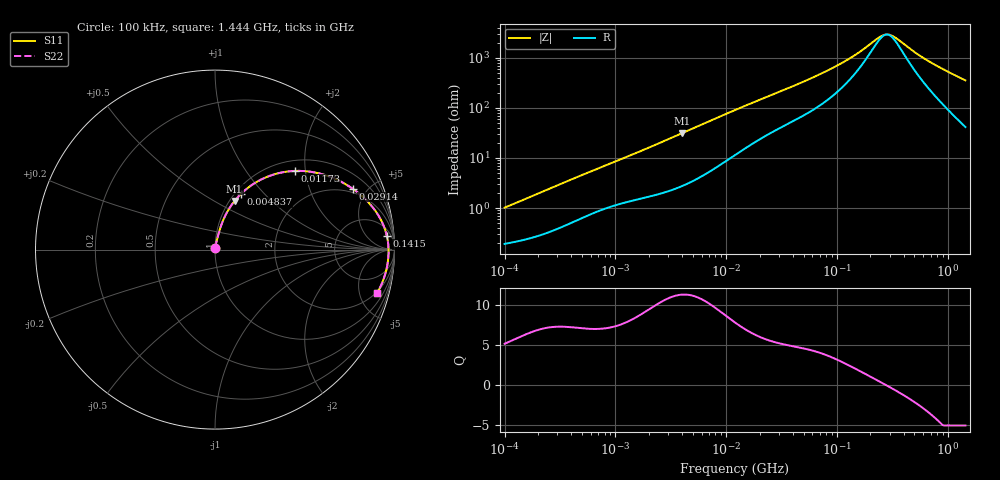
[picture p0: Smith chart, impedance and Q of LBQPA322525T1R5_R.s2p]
! LBQPA322525T1R5_R  S-PARAMETER MODEL  ( General Type )
! Model Generated by TAIYO YUDEN Corporation (http://www.ty-top.com)
! Version 1.0
! TAIYO YUDEN Control No. 191025NI43SB-FBB
! Copyright(c) 2019 TAIYO YUDEN CO.,LTD. All Rights Reserved.
! Product Description (link to TY-COMPAS)
! https://ds.yuden.co.jp/TYCOMPAS/or/detail?pn=LBQPA322525T1R5MR&u=M
! Products Name : Inductors
! Characteristics :
!  Inductance : 1.5 uH , SRF(min) : 220 MHz , DC Resistance(max) : 0.078 Ohm
!  Rated Current : Saturation :2000 mA , Temp Rise : 1000 mA (20 degC)
!  Case Size : 3.2 x 2.5 / 0.126 x 0.098 [mm/inch] , Thickness : 2.5 / 0.098 [mm/inch]
!  (Conditions: Temperature = 25 degC , DC Bias Current/Voltage = 0A / 0V)
! External Node Assignments :
!  1  o---GGG---o  2
! GND o---------o GND
! Frequency Range : 0.1MHz  -  1443.872596MHz  [ 402 STEP ]
# MHz S RI R 50
! Freq[MHz].  S11 Real  S11 Imag  S21 Real  S21 Imag  S12 Real  S12 Imag  S22 Real  S22 Imag
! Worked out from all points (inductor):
!   401 points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, 100 kHz to 1.444 GHz, reference 50 ohm
!   read as one part in series: L = 1.57 uH near 104.9 kHz
!   highest Q = 11.4 at 3.994 MHz (marker M1), where L = 1.24 uH
!   self-resonance near 281.6 MHz
!   S11 on the Smith chart (normalised r, x): 100 kHz: 1.00, +0.02; 4.837 MHz: 1.07, +0.75; 11.73 MHz: 1.22, +1.76; 29.14 MHz: 1.75, +4.00; 141.5 MHz: 10, +20; 1.444 GHz: 1.83, -7.06
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0.1  0.00202 0.01  0.998 -0.01  0.998 -0.01  0.00202 0.01
0.497418  0.00827 0.0445  0.9917 -0.0445  0.9917 -0.0445  0.00827 0.0445
1.235596  0.0228 0.0986  0.9772 -0.0986  0.9772 -0.0986  0.0228 0.0986
2.474242  0.0538 0.1823  0.9462 -0.1823  0.9462 -0.1823  0.0538 0.1823
3.994097  0.1091 0.2709  0.8909 -0.2709  0.8909 -0.2709  0.1091 0.2709
4.837369  0.1458 0.3113  0.8542 -0.3113  0.8542 -0.3113  0.1458 0.3113
7.267569  0.2601 0.3919  0.7399 -0.3919  0.7399 -0.3919  0.2601 0.3919
11.73183  0.4474 0.4384  0.5526 -0.4384  0.5526 -0.4384  0.4474 0.4384
12.01613  0.4573 0.4387  0.5427 -0.4387  0.5427 -0.4387  0.4573 0.4387
17.62567  0.6099 0.4163  0.3901 -0.4163  0.3901 -0.4163  0.6099 0.4163
29.1421  0.7666 0.3393  0.2334 -0.3393  0.2334 -0.3393  0.7666 0.3393
59.77031  0.8993 0.2075  0.1007 -0.2075  0.1007 -0.2075  0.8993 0.2075
96.48548  0.9412 0.1291  0.0588 -0.1291  0.0588 -0.1291  0.9412 0.1291
141.5282  0.9575 0.0769  0.0425 -0.0769  0.0425 -0.0769  0.9575 0.0769
245.48  0.9664 0.0145  0.0336 -0.0145  0.0336 -0.0145  0.9664 0.0145
270.1539  0.9669 0.00438  0.0331 -0.00438  0.0331 -0.00438  0.9669 0.00438
297.308  0.9671 -0.00575  0.0329 0.00575  0.0329 0.00575  0.9671 -0.00575
343.2413  0.967 -0.0211  0.033 0.0211  0.033 0.0211  0.967 -0.0211
491.566  0.9639 -0.0619  0.0361 0.0619  0.0361 0.0619  0.9639 -0.0619
671.0681  0.957 -0.1029  0.043 0.1029  0.043 0.1029  0.957 -0.1029
1008.2  0.9375 -0.1696  0.0625 0.1696  0.0625 0.1696  0.9375 -0.1696
1443.873  0.9022 -0.2439  0.0978 0.2439  0.0978 0.2439  0.9022 -0.2439
